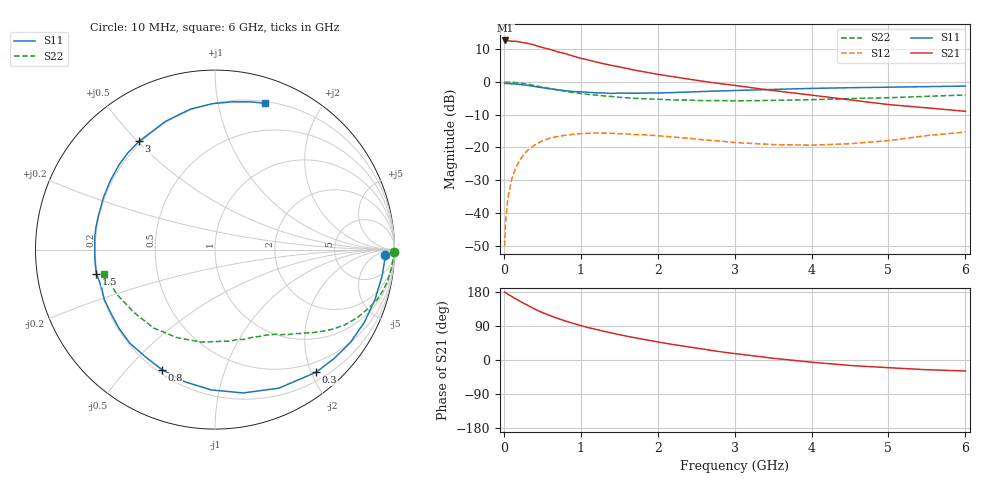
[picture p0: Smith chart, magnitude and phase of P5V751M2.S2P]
! SIEMENS Small Signal Semiconductors
! BFP183
! Si NPN RF Bipolar Junction Transistor in SOT143
! VCE = 0.75 V  IC = 1.2 mA
! Common Emitter S-Parameters:  March  1996
# GHz  S  MA  R  50
!  f  S11  S21  S12  S22
! GHz  MAG  ANG  MAG  ANG  MAG  ANG  MAG  ANG
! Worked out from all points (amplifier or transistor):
!   36 points, 10 MHz to 6 GHz, reference 50 ohm
!   highest |S21| = 12.6 dB at 20 MHz (marker M1)
!   |S21| within 3 dB of that: start of sweep to 638.5 MHz
!   unconditionally stable (mu >= 1): 2.268 GHz to end of sweep
!   at 250 MHz: K = 0.12, MSG = 17.2 dB, |S12| = -22.5 dB
!   at 1.4 GHz: K = 0.61, MSG = 10.4 dB, |S12| = -15.7 dB
!   at 6 GHz: K = 1.22, MAG = 0.3 dB, |S12| = -15.3 dB
!   S11 on the Smith chart (normalised r, x): 10 MHz: 29, -16; 300 MHz: 0.33, -2.08; 800 MHz: 0.22, -0.63; 1.5 GHz: 0.20, -0.10; 3 GHz: 0.19, +0.51; 6 GHz: 0.22, +1.38
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0.01  0.949 -1.7  4.219 179.1  0.0031 86.8  0.9997 -0.7
0.02  0.9467 -3.7  4.285 178.2  0.0066 89.1  0.9904 -1.4
0.05  0.9429 -8.9  4.265 173.9  0.0159 84.8  0.9929 -3.5
0.1  0.934 -17.3  4.165 168.0  0.032 78.6  0.9849 -7.2
0.15  0.9256 -25.9  4.171 161.9  0.0473 74.0  0.976 -10.8
0.2  0.915 -34.3  4.078 156.1  0.0618 69.4  0.9612 -14.1
0.3  0.8855 -50.5  3.9 145.4  0.0877 60.4  0.9218 -20.2
0.4  0.85 -65.3  3.641 134.6  0.1088 51.5  0.8783 -25.7
0.5  0.8139 -78.9  3.344 125.2  0.1253 44.1  0.8337 -30.3
0.6  0.782 -91.6  3.137 117.2  0.1381 37.7  0.7922 -34.0
0.7  0.7551 -103.0  2.875 109.8  0.1468 31.9  0.7507 -37.3
0.8  0.7311 -113.9  2.692 102.8  0.1531 26.7  0.7172 -40.1
0.9  0.7118 -123.1  2.475 96.8  0.1582 22.3  0.6869 -42.5
1.1  0.6918 -140.7  2.154 85.3  0.1637 14.7  0.6424 -46.8
1.5  0.6742 -168.6  1.692 66.8  0.1615 3.4  0.5807 -54.3
1.8  0.6737 173.7  1.438 55.0  0.1561 -2.1  0.5536 -59.5
2.2  0.6864 154.6  1.199 40.8  0.1437 -7.5  0.5299 -67.5
3  0.7367 125.0  0.883 17.0  0.1184 -9.5  0.5123 -85.8
3.5  0.7659 111.1  0.736 4.6  0.1102 -4.7  0.5212 -98.4
4.5  0.8138 90.7  0.53 -14.4  0.1136 8.7  0.5552 -128.2
5.5  0.8457 76.9  0.401 -25.7  0.1513 15.4  0.601 -155.5
6  0.862 71.0  0.355 -28.9  0.1713 13.2  0.6308 -167.8
